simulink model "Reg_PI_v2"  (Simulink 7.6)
settings: Solver=ode45  StartTime=0.0  StopTime=10.0  RelTol=1e-3
InitFcn:
  | Kp=0.01;
  | R1=10e3;
  | R2=Kp*R1;
  | 
  | Ti=0.001;
  | C=Ti/R2;
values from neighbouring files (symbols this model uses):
  R = 1e3    (= 1000)    [oscillateur_dephasage.m]    (also in Calcul_Ampl_phase_A.m = 1; circuit_RLC_parallele_.m = 4; symbolique_circuit_RC.m = 4; parametres.m = 4)
libraries: fl_lib x4, elec_lib x1

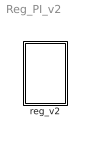
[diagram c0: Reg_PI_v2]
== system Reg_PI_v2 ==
  reg_v2 : Subsystem

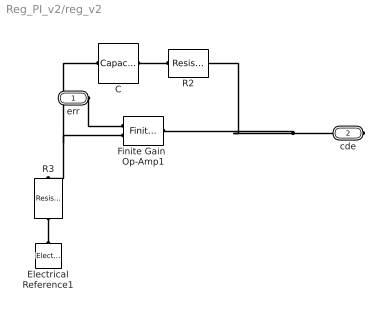
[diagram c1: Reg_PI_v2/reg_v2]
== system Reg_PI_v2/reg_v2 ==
  C : fl_lib/Electrical/Electrical Elements/Capacitor  DialogController=NetworkEngine.DynNeDlgSource  SystemSampleTime=-1  c=C F  v0=0 V  r=1e-6 Ohm  g=0 1/Ohm  i_Log=off  v_Log=off  vc_Log=off  LocalVarNames=|i|v|vc  LocalVarDescs=|i|v|Internal variable for voltage across capacitor term  LocalVarLogging=[0 0 0]
  Electrical Reference1 : fl_lib/Electrical/Electrical Elements/Electrical Reference  DialogController=NetworkEngine.DynNeDlgSource  SystemSampleTime=-1  i_Log=off  LocalVarNames=|i  LocalVarDescs=|i  LocalVarLogging=[]
  Finite Gain  Op-Amp1 : elec_lib/Integrated Circuits/Finite Gain Op-Amp  DialogController=NetworkEngine.DynNeDlgSource  SystemSampleTime=-1  A=1000  Rin=1e+6 Ohm  Rout=100 Ohm  Vmin=-15 V  Vmax=15 V  LocalVarLogging=[]
  R2 : fl_lib/Electrical/Electrical Elements/Resistor  DialogController=NetworkEngine.DynNeDlgSource  SystemSampleTime=-1  R=R Ohm  i_Log=off  v_Log=off  LocalVarNames=|current|voltage|power  LocalVarDescs=|Resistor current (A)|Voltage across resistor (V)|Power (W)  LocalVarLogging=[0 0 0]
  R3 : fl_lib/Electrical/Electrical Elements/Resistor  DialogController=NetworkEngine.DynNeDlgSource  SystemSampleTime=-1  R=R Ohm  i_Log=off  v_Log=off  LocalVarNames=|current|voltage|power  LocalVarDescs=|Resistor current (A)|Voltage across resistor (V)|Power (W)  LocalVarLogging=[0 0 0]
  err : PMIOPort  Port=1  Side=Left
  cde : PMIOPort  Port=2  Side=Right
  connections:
  C/LConn1 -- R3/RConn1 -- Finite Gain  Op-Amp1/LConn2
  C/RConn1 -- R2/LConn1
  R3/LConn1 -- Electrical Reference1/LConn1
  err/RConn1 -- Finite Gain  Op-Amp1/LConn1
  cde/RConn1 -- R2/RConn1 -- Finite Gain  Op-Amp1/RConn1
